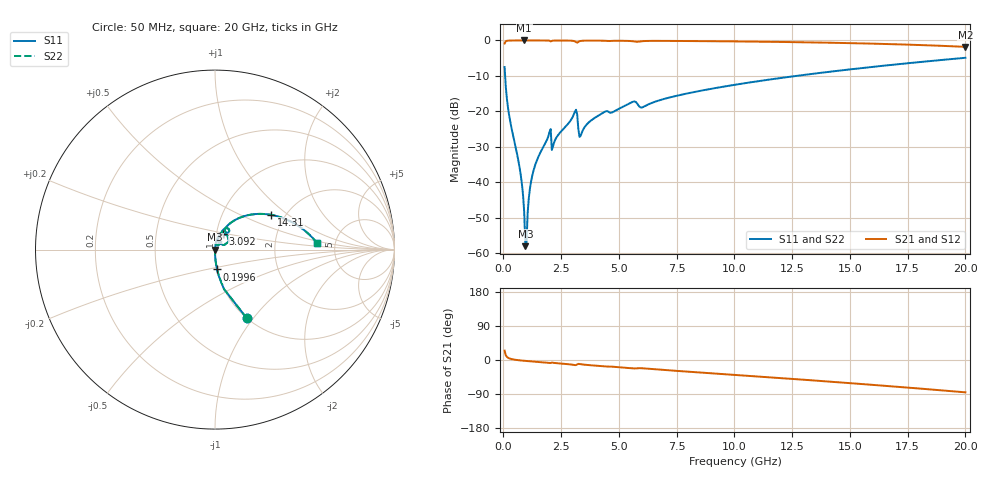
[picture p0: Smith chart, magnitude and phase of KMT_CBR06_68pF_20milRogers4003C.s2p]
! Data measured by Modelithics Inc. support@modelithics.com 813-866-6335
! KEMET CBR0603 68pF, Pad Width= 0.851mm, Pad Length= 0.64mm, Pad Gap= 0.62mm, 20mil Rogers 4003C substrate Data, January 2022
# hz S ma R 50
! 2 Port Network Data from SP1.SP block
! freq  magS11  angS11  magS21  angS21  magS12  angS12  magS22  angS22
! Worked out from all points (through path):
!   401 points, 50 MHz to 20 GHz, reference 50 ohm
!   highest |S21| = 0.00 dB at 897.9 MHz (marker M1); lowest = -1.8 dB at 20 GHz (marker M2)
!   group delay of S21, straight-line fit = 12 ps
!   lowest |S11| = -58.0 dB at 947.8 MHz (marker M3), VSWR 1.00, Z = 50 - j0.122 ohm
!   |S11| at or under -10 dB: 72.82 MHz to 12.67 GHz (12.6 GHz wide, 198 % of centre)
!   |S22| runs from -58.0 to -4.9 dB; largest |S21 - S12| = 0
!   S11 on the Smith chart (normalised r, x): 50 MHz: 1.00, -0.93; 199.6 MHz: 1.00, -0.22; 3.092 GHz: 1.08, +0.19; 14.31 GHz: 1.70, +0.76; 20 GHz: 3.60, +0.40
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5e7  0.4215 -65.2  0.9066 24.8  0.9066 24.8  0.4215 -65.2
1.99625e8  0.1112 -84.0  0.9936 5.9  0.9936 5.9  0.1112 -84.0
6.98375e8  0.01623 -89.6  0.9995 -0.9  0.9995 -0.9  0.01623 -89.6
7.98125e8  0.009579 -89.3  0.9996 -1.5  0.9996 -1.5  0.009579 -89.3
8.97875e8  0.003845 -86.2  0.9996 -2.1  0.9996 -2.1  0.003845 -86.2
9.4775e8  0.001265 -73.8  0.9996 -2.4  0.9996 -2.4  0.001265 -73.8
1.0475e9  0.003707 80.5  0.9995 -2.9  0.9995 -2.9  0.003707 80.5
1.14725e9  0.008203 83.5  0.9995 -3.4  0.9995 -3.4  0.008203 83.5
1.247e9  0.01244 83.9  0.9994 -3.9  0.9994 -3.9  0.01244 83.9
1.54625e9  0.02435 83.3  0.9991 -5.4  0.9991 -5.4  0.02435 83.3
1.94525e9  0.04491 78.6  0.9959 -7.6  0.9959 -7.6  0.04491 78.6
2.194625e9  0.03673 77.9  0.9964 -7.7  0.9964 -7.7  0.03673 77.9
3.092375e9  0.09899 62.4  0.9711 -13.4  0.9711 -13.4  0.09899 62.4
3.391625e9  0.05014 66.9  0.9886 -11.5  0.9886 -11.5  0.05014 66.9
4.389125e9  0.09908 69.3  0.9884 -16.9  0.9884 -16.9  0.09908 69.3
5.586125e9  0.136 61.6  0.9756 -22.1  0.9756 -22.1  0.136 61.6
6.73325e9  0.1429 63.2  0.9861 -25.4  0.9861 -25.4  0.1429 63.2
1.0025e10  0.2376 50.3  0.9691 -39.3  0.9691 -39.3  0.2376 50.3
1.336662e10  0.3381 35.9  0.9382 -53.7  0.9382 -53.7  0.3381 35.9
1.431425e10  0.3685 31.7  0.9264 -57.9  0.9264 -57.9  0.3685 31.7
1.670825e10  0.4493 20.5  0.8887 -69.0  0.8887 -69.0  0.4493 20.5
2e10  0.5695 3.8  0.8123 -85.3  0.8123 -85.3  0.5695 3.8
